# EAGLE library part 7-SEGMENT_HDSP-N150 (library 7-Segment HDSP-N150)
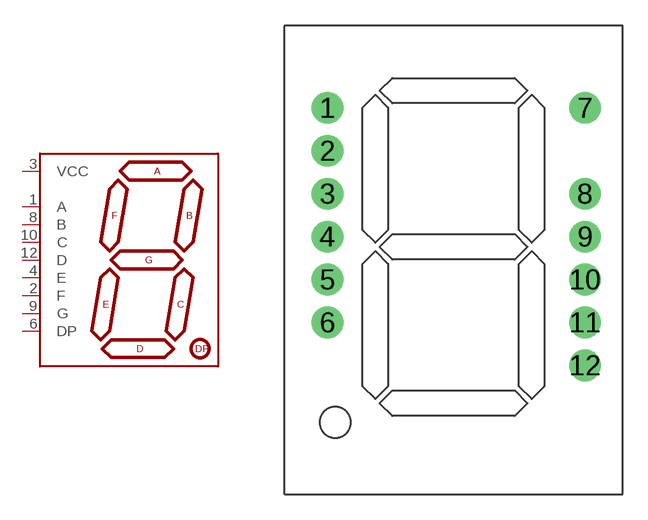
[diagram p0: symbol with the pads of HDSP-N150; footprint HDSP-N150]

Designator prefix -

## 7-SEGMENT_HDSP-N150  [HDSP-N150]
1  A
2  F
3  VCC
4  E
6  DP
8  B
9  G
10  C
12  D

## Footprint HDSP-N150 (pad centres in mm)
drill 1.016 pad 1.88: 1 2.54,22.86; 2 2.54,20.32; 3 2.54,17.78; 4 2.54,15.24; 5 2.54,12.7; 6 2.54,10.16; 7 17.78,22.86; 8 17.78,17.78; 9 17.78,15.24; 10 17.78,12.7; 11 17.78,10.16; 12 17.78,7.62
